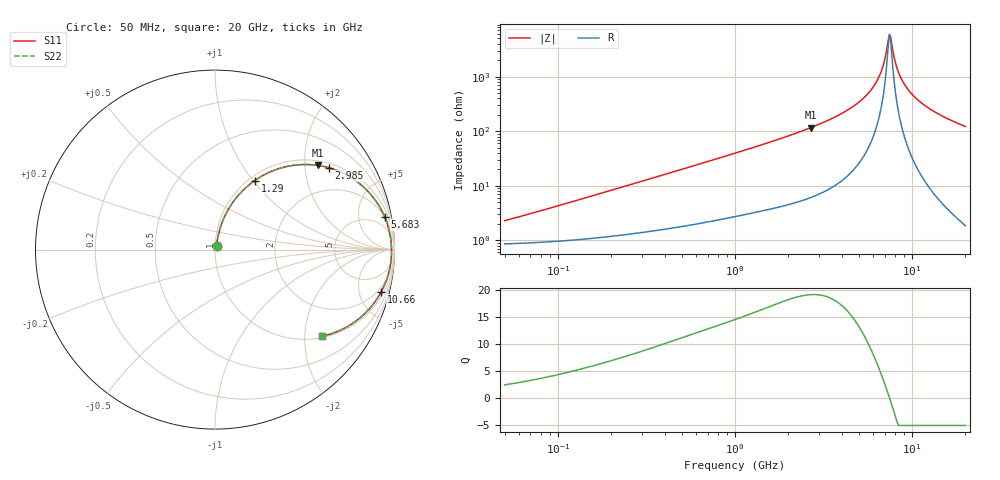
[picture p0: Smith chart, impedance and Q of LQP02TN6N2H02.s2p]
!Murata Part Number: LQP02TN6N2H02
!These Parameters are Measured in Series Mode Connection
!  o--[Z]--o
!Port1  Port2
!  o-------o
!Freq. Start=50[MHz] Stop=20[GHz], 401[Steps]
# Hz S RI R 50
!Freq.(Hz) S11(Real) S11(Imag) S21(Real) S21(Imag) S12(Real) S12(Imag) S22(Real) S22(Imag)
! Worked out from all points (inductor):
!   401 points, 50 MHz to 20 GHz, reference 50 ohm
!   read as one part in series: L = 6.7 nH near 63.54 MHz
!   highest Q = 19.1 at 2.687 GHz (marker M1), where L = 6.9 nH
!   self-resonance near 7.442 GHz
!   S11 on the Smith chart (normalised r, x): 50 MHz: 1.02, +0.04; 1.29 GHz: 1.06, +1.02; 2.985 GHz: 1.14, +2.68; 5.683 GHz: 2, +10; 10.66 GHz: 1.42, -7.70; 20 GHz: 1.04, -2.43
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5e7  0.00898 0.0209  0.991 -0.0209  0.991 -0.0209  0.00898 0.0209
1.364002e8  0.0134 0.0552  0.9866 -0.0552  0.9866 -0.0552  0.0134 0.0552
3.721004e8  0.036 0.1418  0.964 -0.1418  0.964 -0.1418  0.036 0.1418
1e9  0.1515 0.3257  0.8485 -0.3257  0.8485 -0.3257  0.1515 0.3257
1.289994e9  0.2218 0.385  0.7782 -0.385  0.7782 -0.385  0.2218 0.385
2.687447e9  0.5729 0.4691  0.4271 -0.4691  0.4271 -0.4691  0.5729 0.4691
2.728004e9  0.5818 0.4677  0.4182 -0.4677  0.4182 -0.4677  0.5818 0.4677
2.98453e9  0.6356 0.4557  0.3644 -0.4557  0.3644 -0.4557  0.6356 0.4557
4.34015e9  0.8433 0.3335  0.1567 -0.3335  0.1567 -0.3335  0.8433 0.3335
5.683258e9  0.9451 0.1828  0.0549 -0.1828  0.0549 -0.1828  0.9451 0.1828
6.217679e9  0.9656 0.1248  0.0344 -0.1248  0.0344 -0.1248  0.9656 0.1248
6.601595e9  0.975 0.0848  0.025 -0.0848  0.025 -0.0848  0.975 0.0848
6.905011e9  0.9799 0.0542  0.0201 -0.0542  0.0201 -0.0542  0.9799 0.0542
7.331367e9  0.9833 0.0131  0.0167 -0.0131  0.0167 -0.0131  0.9833 0.0131
7.442007e9  0.9836 0.00281  0.0164 -0.00281  0.0164 -0.00281  0.9836 0.00281
7.668323e9  0.9836 -0.0179  0.0164 0.0179  0.0164 0.0179  0.9836 -0.0179
8.141811e9  0.9808 -0.0591  0.0192 0.0591  0.0192 0.0591  0.9808 -0.0591
8.644534e9  0.9745 -0.1  0.0255 0.1  0.0255 0.1  0.9745 -0.1
9.457416e9  0.9586 -0.1601  0.0414 0.1601  0.0414 0.1601  0.9586 -0.1601
1.066139e10  0.9257 -0.2362  0.0743 0.2362  0.0743 0.2362  0.9257 -0.2362
1.396067e10  0.8088 -0.3795  0.1912 0.3795  0.1912 0.3795  0.8088 -0.3795
2e10  0.5955 -0.4832  0.4045 0.4832  0.4045 0.4832  0.5955 -0.4832
